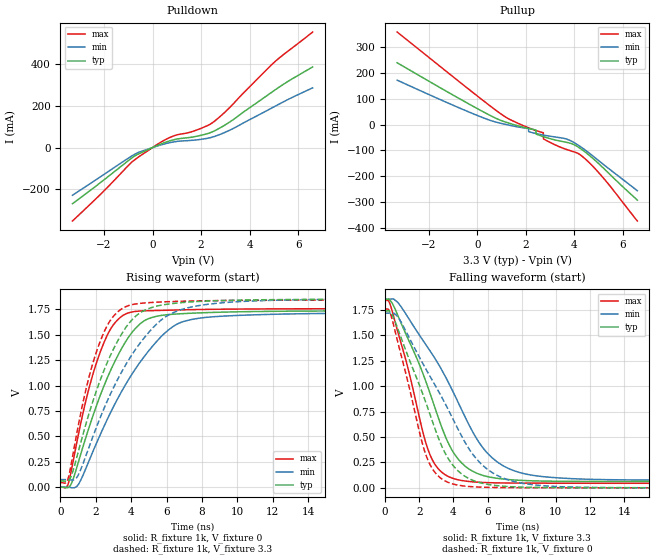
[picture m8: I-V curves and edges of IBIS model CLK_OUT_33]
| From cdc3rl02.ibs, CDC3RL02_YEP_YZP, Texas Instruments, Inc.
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[Model]   CLK_OUT_33
Model_type  Output
Vref =   1.8
Rref =   1M
Cref =   30p
Vmeas =   0.9
| variable   typ   min   max
C_comp   38.02pF   22.91pF   52.31pF
| C_pullup   32.87pF   22.91pF   36.95pF
| C_pulldown   43.18pF   36.02pF   52.31pF
[Temperature Range]   40   100   -40
| Ambient temperature   25   85   -40
[Voltage range]   3.3   3   3.6
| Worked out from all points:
|   slope of the pulldown table from 0 to 0.495 V, typ, clamps not added: 20.8 ohm
|   slope of the pullup table from 0 to 0.495 V, typ, clamps not added: 20 ohm
|   rising waveform, R_fixture 1k, V_fixture 0: 20-80 % time 2.35ns typ, 3.32ns min, 1.6ns max; typ from 0 V to 1.74 V
|   falling waveform, R_fixture 1k, V_fixture 3.3: 20-80 % time 2.5ns typ, 3.55ns min, 1.63ns max; typ from 1.85 V to 0.061 V
|   rising waveform, R_fixture 1k, V_fixture 3.3: 20-80 % time 2.29ns typ, 3.17ns min, 1.57ns max; typ from 0.061 V to 1.85 V
|   falling waveform, R_fixture 1k, V_fixture 0: 20-80 % time 2.37ns typ, 3.35ns min, 1.55ns max; typ from 1.74 V to 0 V
[Pulldown]
| CLK_OUT_33
|   Voltage   I(typ)   I(min)   I(max)
-3.3V     -268.6mA   -228.1mA   -351.4mA
-2.035V   -157.6mA   -131.1mA   -211.1mA
-910mV    -54.84mA   -44.28mA   -75.62mA
-615mV    -32.69mA   -25.02mA   -48.26mA
220mV     11.25mA    8.32mA     16.92mA
670mV     30.61mA    22.44mA    45.91mA
1V        40.48mA    29.24mA    60.52mA
1.74V     52.26mA    35.79mA    80.58mA
2.475V    75.76mA    50.31mA    119.4mA
3.22V     125.2mA    85.21mA    196.3mA
5.03V     274.2mA    196.5mA    409.3mA
6.6V      386mA      285.8mA    552.8mA
[Pullup]
| CLK_OUT_33
|   Voltage   I(typ)   I(min)   I(max)
-3.3V     238.7mA    171.5mA    357.4mA
1.1V      11.83mA    2.15mA     33.25mA
2.115V    -15.11mA   -15.34mA   -12.36mA
2.12V     -15.22mA   -27.44mA   -12.55mA
2.42V     -20.86mA   -34.56mA   -22.85mA
2.425V    -36.77mA   -34.68mA   -23mA
2.725V    -46.48mA   -40.62mA   -31.67mA
2.73V     -46.64mA   -40.7mA    -55.31mA
3.66V     -68.26mA   -55.36mA   -95.42mA
4.3V      -95.62mA   -88.19mA   -120.7mA
5.23V     -170.8mA   -156mA     -209.6mA
6.6V      -291.8mA   -255.7mA   -372.5mA
[Ramp]
| CLK_OUT_33
| variable   typ   min   max
dV/dt_r   1.05/2.36E-09   1.03/3.33E-09   1.06/1.60E-09
dV/dt_f   1.08/2.51E-09   1.07/3.55E-09   1.08/1.63E-09
R_load = 1k
[Rising Waveform]
| CLK_OUT_33
R_fixture =   1k
C_fixture =   0
L_fixture =   0
V_fixture =   0
V_fixture_min = 0
V_fixture_max = 0
|   Time   V(typ)   V(min)   V(max)
0s        9.559nV    28.61nV    2.329nV
461ps     170.2uV    -574uV     46.06mV
1.029ns   256.5mV    31.82mV    530.5mV
1.685ns   624.2mV    289.1mV    1.02V
2.421ns   980mV      583.2mV    1.406V
3.093ns   1.244V     824.2mV    1.62V
3.949ns   1.501V     1.087V     1.721V
6.125ns   1.699V     1.55V      1.742V
8.141ns   1.717V     1.67V      1.749V
37.43ns   1.737V     1.717V     1.757V
[Falling Waveform]
| CLK_OUT_33
R_fixture =   1k
C_fixture =   0
L_fixture =   0
V_fixture =   3.3
V_fixture_min = 3
V_fixture_max = 3.6
|   Time   V(typ)   V(min)   V(max)
0s        1.851V     1.854V     1.842V
381ps     1.823V     1.857V     1.757V
885ps     1.638V     1.791V     1.45V
2.557ns   964.8mV    1.365V     355.9mV
3.189ns   655.1mV    1.197V     174mV
4.125ns   316.3mV    893.6mV    85.3mV
5.253ns   152.7mV    514mV      57.49mV
6.109ns   106.6mV    321.1mV    50.69mV
8.765ns   68.43mV    120.2mV    46.02mV
37.43ns   61.43mV    75.05mV    44.64mV
[Rising Waveform]
| CLK_OUT_33
R_fixture =   1k
C_fixture =   0
L_fixture =   0
V_fixture =   3.3
V_fixture_min = 3
V_fixture_max = 3.6
|   Time   V(typ)   V(min)   V(max)
0s        61.44mV    75.06mV    44.65mV
421ps     61.01mV    74.97mV    78.45mV
949ps     311mV      102.8mV    553.2mV
1.573ns   700.4mV    374.3mV    1.055V
2.261ns   1.059V     690.4mV    1.441V
2.941ns   1.34V      958.9mV    1.671V
3.981ns   1.635V     1.288V     1.794V
5.981ns   1.799V     1.681V     1.825V
8.829ns   1.835V     1.81V      1.836V
37.43ns   1.851V     1.853V     1.842V
[Falling Waveform]
| CLK_OUT_33
R_fixture =   1k
C_fixture =   0
L_fixture =   0
V_fixture =   0
V_fixture_min = 0
V_fixture_max = 0
|   Time   V(typ)   V(min)   V(max)
0s        1.737V     1.717V     1.757V
389ps     1.706V     1.721V     1.669V
901ps     1.49V      1.639V     1.327V
2.421ns   821.5mV    1.158V     309.4mV
3.061ns   517.2mV    969.1mV    124.8mV
4.005ns   215.1mV    666.5mV    36.49mV
4.965ns   86.78mV    370.5mV    12.55mV
5.877ns   38.33mV    198mV      5.492mV
8.589ns   4.931mV    31.87mV    1.323mV
37.43ns   -9.786uV   -13.07uV   -6.671uV
